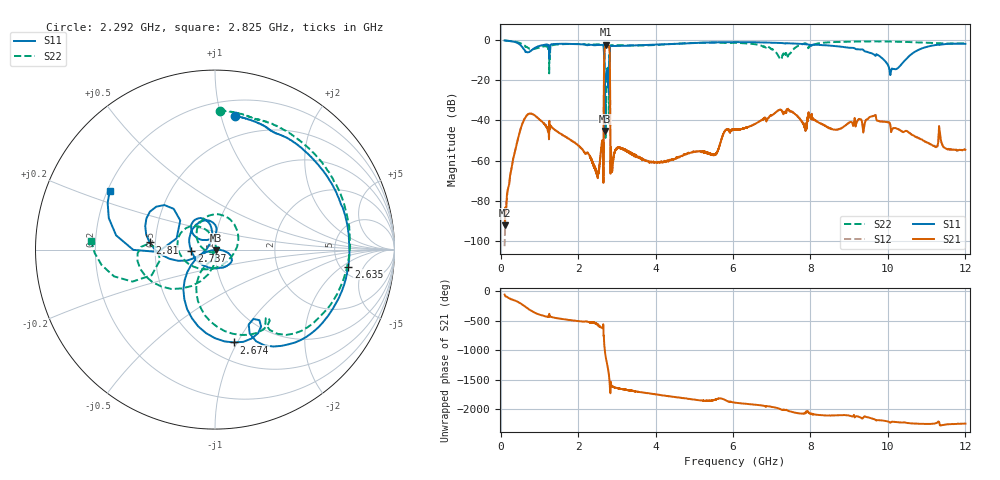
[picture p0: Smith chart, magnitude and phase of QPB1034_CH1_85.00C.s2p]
! TDS: k:\Engsetup\Winsaw\QPB1034_ALL
! Channel 1
! Ports=1 2
! seg 1=100.000000 1100.000000 51
! seg 2=1101.000000 1301.000000 201
! seg 3=1302.000000 2302.000000 101
! seg 4=2303.000000 3503.000000 1201
! seg 5=3504.000000 5204.000000 171
! seg 6=5205.000000 6405.000000 1201
! seg 7=6406.000000 8506.000000 211
! seg 8=8507.000000 12007.000000 176
! Points=3313
! FailCode=0
! Topology=ALL_SE(12)
!VNA Cal loaded =QPB1034_ALL_85C
!PS1(V)= 5.000
!PS(mA)= 0.280
!PS2(V)= 0.630
!PS(mA)= -0.003
!PS3(V)= 0.630
!PS(mA)= -0.002
!PS4(V)= 1.170
!PS(mA)= -0.001
!Temp (C)= 85.00
# MHz S DB R 50
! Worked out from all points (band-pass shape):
!   3313 points, 100 MHz to 12.01 GHz, reference 50 ohm
!   highest |S21| = -2.47 dB at 2.728 GHz (marker M1); lowest = -92.0 dB at 100 MHz (marker M2)
!   |S21| within 3 dB of the highest: 2.682 GHz to 2.811 GHz (128.8 MHz wide, 4.69 % of centre)
!   lowest |S11| = -45.2 dB at 2.69 GHz (marker M3), VSWR 1.01, Z = 50.5 - j0.2 ohm
!   |S11| at or under -10 dB: 2.681 GHz to 2.808 GHz (127.3 MHz wide, 4.64 % of centre); 2.817086 GHz to 2.819989 GHz (2.903 MHz wide, 0.103 % of centre); 9.905 GHz to 10.45 GHz (550 MHz wide, 5.4 % of centre)
!   |S22| runs from -48.7 to -0.3 dB; largest |S21 - S12| = 0.0038
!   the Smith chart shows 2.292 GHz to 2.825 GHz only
!   S11 on the Smith chart (normalised r, x): 2.292 GHz: 0.33, +1.11; 2.635 GHz: 5.84, -2.50; 2.674 GHz: 0.68, -0.97; 2.737 GHz: 0.77, -0.01; 2.81 GHz: 0.46, +0.04; 2.825 GHz: 0.21, +0.25
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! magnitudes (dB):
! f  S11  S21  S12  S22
! 100 MHz  -0.3  -92.0  -102.5  -0.3
! 240 MHz  -0.6  -67.7  -67.9  -0.6
! 500 MHz  -2.4  -45.1  -45.2  -1.6
! 1.1 GHz  -2.6  -41.3  -41.3  -3.2
! 2.292 GHz  -2.5  -57.2  -57.5  -2.2
! 2.434 GHz  -2.7  -63.4  -64.0  -2.3
! 2.635 GHz  -2.5  -51.0  -51.0  -2.5
! 2.649 GHz  -2.7  -50.9  -51.1  -2.7
! 2.674 GHz  -5.5  -9.5  -9.4  -5.8
! 2.69 GHz  -45.2  -3.7  -3.7  -20.8
! 2.711 GHz  -18.9  -2.8  -2.7  -34.2
! 2.728 GHz  -19.2  -2.5  -2.5  -29.8
! 2.737 GHz  -17.5  -2.6  -2.6  -19.6
! 2.81 GHz  -8.7  -5.1  -5.1  -8.8
! 2.825 GHz  -3.4  -22.1  -22.1  -3.2
! 2.848 GHz  -3.1  -53.9  -53.9  -2.7
! 2.877 GHz  -3.1  -64.8  -65.0  -2.7
! 3.052 GHz  -3.1  -53.4  -53.4  -2.7
! 5.406 GHz  -1.3  -56.6  -56.6  -1.4
! 7.306 GHz  -1.7  -37.0  -36.9  -6.7
! 10.17 GHz  -14.5  -43.8  -43.9  -0.9
! 12.01 GHz  -2.0  -54.6  -54.7  -1.8
